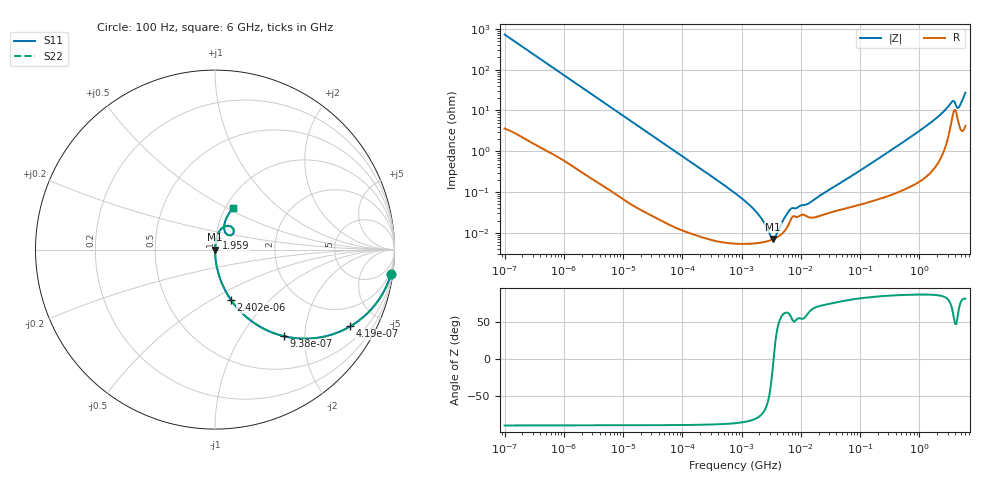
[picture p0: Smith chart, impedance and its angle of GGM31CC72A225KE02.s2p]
!Murata Part Number: GGM31CC72A225KE02
!These Parameters are Measured in Series Mode Connection
!Data Generated on Jun 19, 2026
!  o--ll--o
!Port1  Port2
!  o------o
!Operation Temp=25[degC], DC Bias Voltage=0[V]
!Freq. Start=100[Hz] Stop=6[GHz] 401[Steps]
# Hz S RI R 50
!Freq.(Hz) S11(Real) S11(Imag) S21(Real) S21(Imag) S12(Real) S12(Imag) S22(Real) S22(Imag)
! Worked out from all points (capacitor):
!   401 points, 100 Hz to 6 GHz, reference 50 ohm
!   read as one part in series: C = 2.17 uF near 109 Hz
!   lowest |Z| = 7.02 mohm at 3.394 MHz (marker M1)
!   series resonance near 3.469 MHz, so ESL is about 970 pH
!   S11 on the Smith chart (normalised r, x): 100 Hz: 1, -15; 419 Hz: 1.02, -3.51; 938 Hz: 1.01, -1.57; 2.402 kHz: 1.01, -0.62; 1.959 GHz: 1.01, +0.13; 6 GHz: 1.08, +0.54
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100  0.981 -0.134  0.019 0.134  0.019 0.134  0.981 -0.134
224  0.9134 -0.2782  0.0866 0.2782  0.0866 0.2782  0.9134 -0.2782
419  0.7535 -0.4276  0.2465 0.4276  0.2465 0.4276  0.7535 -0.4276
627  0.5795 -0.4899  0.4205 0.4899  0.4205 0.4899  0.5795 -0.4899
938  0.3836 -0.4823  0.6164 0.4823  0.6164 0.4823  0.3836 -0.4823
2008  0.122 -0.3232  0.878 0.3232  0.878 0.3232  0.122 -0.3232
2402  0.0891 -0.2808  0.9109 0.2808  0.9109 0.2808  0.0891 -0.2808
7695  0.0102 -0.096  0.9898 0.096  0.9898 0.096  0.0102 -0.096
40335  0.000561 -0.0187  0.9994 0.0187  0.9994 0.0187  0.000561 -0.0187
774597  5.5e-05 -0.000939  0.9999 0.000939  0.9999 0.000939  5.5e-05 -0.000939
1585629  5.48e-05 -0.000383  0.9999 0.000383  0.9999 0.000383  5.48e-05 -0.000383
2169299  5.79e-05 -0.000216  0.9999 0.000216  0.9999 0.000216  5.79e-05 -0.000216
2837864  6.33e-05 -9.02e-05  0.9999 9.02e-05  0.9999 9.02e-05  6.33e-05 -9.02e-05
3394479  6.95e-05 -9.6e-06  0.9999 9.6e-06  0.9999 9.6e-06  6.95e-05 -9.6e-06
4060267  7.92e-05 7.19e-05  0.9999 -7.19e-05  0.9999 -7.19e-05  7.92e-05 7.19e-05
6644369  0.000196 0.000319  0.9998 -0.000319  0.9998 -0.000319  0.000196 0.000319
1.555665e7  0.000236 0.000556  0.9998 -0.000556  0.9998 -0.000556  0.000236 0.000556
3.124326e8  0.000913 0.00992  0.9991 -0.00992  0.9991 -0.00992  0.000913 0.00992
1.95892e9  0.00874 0.0648  0.9913 -0.0648  0.9913 -0.0648  0.00874 0.0648
3.505958e9  0.0703 0.1328  0.9297 -0.1328  0.9297 -0.1328  0.0703 0.1328
4.586474e9  0.0574 0.0943  0.9426 -0.0943  0.9426 -0.0943  0.0574 0.0943
6e9  0.1009 0.2332  0.8991 -0.2332  0.8991 -0.2332  0.1009 0.2332
